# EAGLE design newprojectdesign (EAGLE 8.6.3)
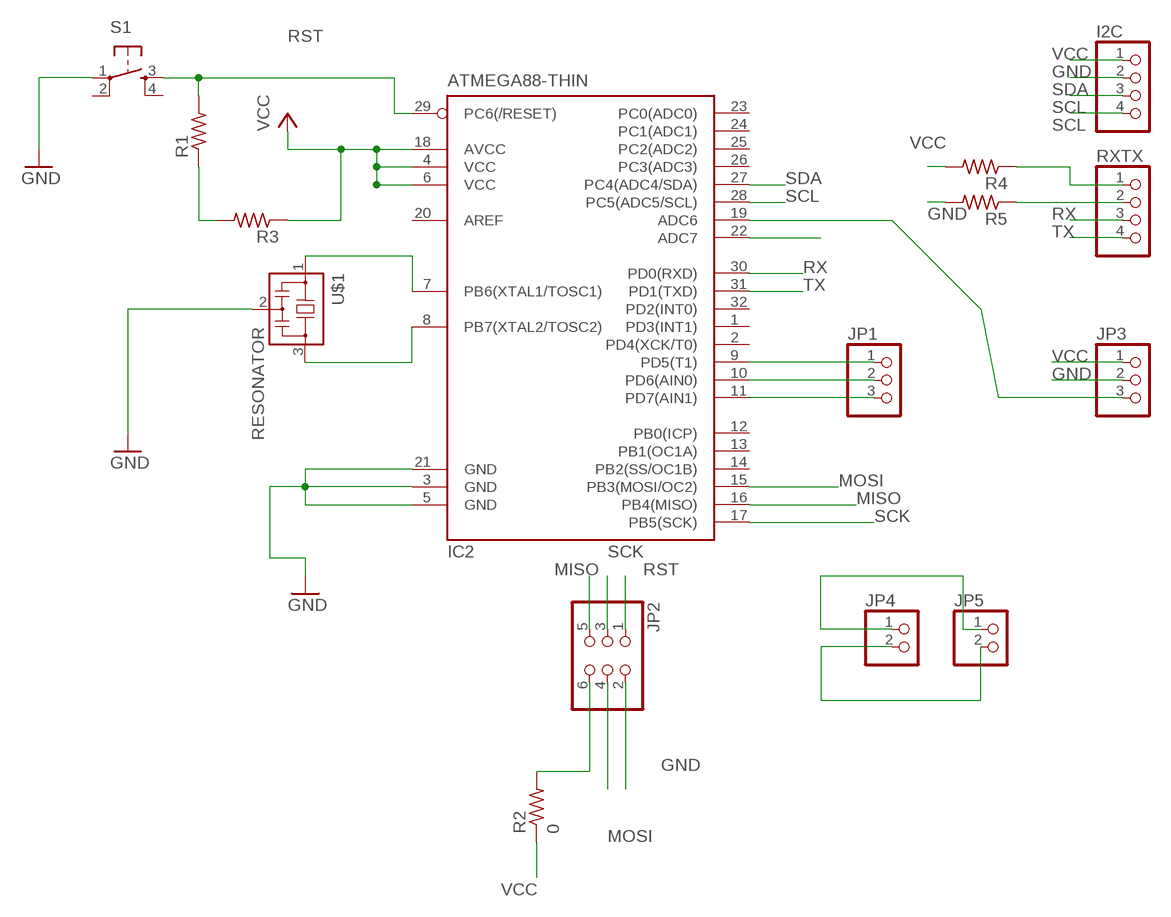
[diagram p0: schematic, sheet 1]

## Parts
I2C  PINHD-1X4  [1X04]
IC2  ATMEGA88-THIN  [TQFP32-08THIN]
JP1  PINHD-1X3  [1X03]
JP2  PINHD-2X3-SMD  [2X03SMD]
JP3  PINHD-1X3  [1X03]
JP4  PINHD-1X2  [1X02]
JP5  PINHD-1X2  [1X02]
R1  RES-US1206FAB  [R1206FAB]
R2  0  RES-US1206FAB  [R1206FAB]
R3  RES-US1206FAB  [R1206FAB]
R4  RES-US1206FAB  [R1206FAB]
R5  RES-US1206FAB  [R1206FAB]
RXTX  PINHD-1X4  [1X04]
S1  6MM_SWITCH6MM_SWITCH  [6MM_SWITCH]
U$1  RESONATOR  [EFOBM]

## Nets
GND: I2C.2 IC2.3(GND) IC2.5(GND) IC2.21(GND) JP2.2 JP3.2 JP4.2 JP5.2 R5.2 S1.1(P) U$1.2
MISO: IC2.16(PB4(MISO)) JP2.5
MOSI: IC2.15(PB3(MOSI/OC2)) JP2.4
N$1: R1.1 R3.2
N$2: IC2.9(PD5(T1)) JP1.1
N$3: JP2.6 R2.2
N$4: IC2.10(PD6(AIN0)) JP1.2
N$5: IC2.11(PD7(AIN1)) JP1.3
N$6: IC2.19(ADC6) JP3.3
N$7: IC2.22(ADC7)
N$8: IC2.8(PB7(XTAL2/TOSC2)) U$1.3
N$9: R4.1 RXTX.1
N$10: R5.1 RXTX.2
N$17: IC2.7(PB6(XTAL1/TOSC1)) U$1.1
RST: IC2.29(PC6(/RESET)) JP2.1 R1.2 S1.3(S)
RX: IC2.30(PD0(RXD)) RXTX.3
SCK: IC2.17(PB5(SCK)) JP2.3
SCL: I2C.4 IC2.28(PC5(ADC5/SCL))
SDA: I2C.3 IC2.27(PC4(ADC4/SDA))
TX: IC2.31(PD1(TXD)) RXTX.4
VCC: I2C.1 IC2.4(VCC) IC2.6(VCC) IC2.18(AVCC) JP3.1 JP4.1 JP5.1 R2.1 R3.1 R4.2
Unconnected: IC2.1(PD3(INT1)) IC2.2(PD4(XCK/T0)) IC2.12(PB0(ICP)) IC2.13(PB1(OC1A)) IC2.14(PB2(SS/OC1B)) IC2.20(AREF) IC2.23(PC0(ADC0)) IC2.24(PC1(ADC1)) IC2.25(PC2(ADC2)) IC2.26(PC3(ADC3)) IC2.32(PD2(INT0)) S1.2(P1) S1.4(S1)

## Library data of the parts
I2C RXTX = pinhead:PINHD-1X4: PIN HEADER
IC2 = fab:ATMEGA88-THIN
JP1 JP3 = adafruit:PINHD-1X3: PIN HEADER
JP2 = fab:PINHD-2X3-SMD: PIN HEADER
JP4 JP5 = pinhead:PINHD-1X2: PIN HEADER
R1-R5 = fab:RES-US: Resistor (US Symbol)
S1 = fab:6MM_SWITCH: OMRON SWITCH
U$1 = fab:RESONATOR

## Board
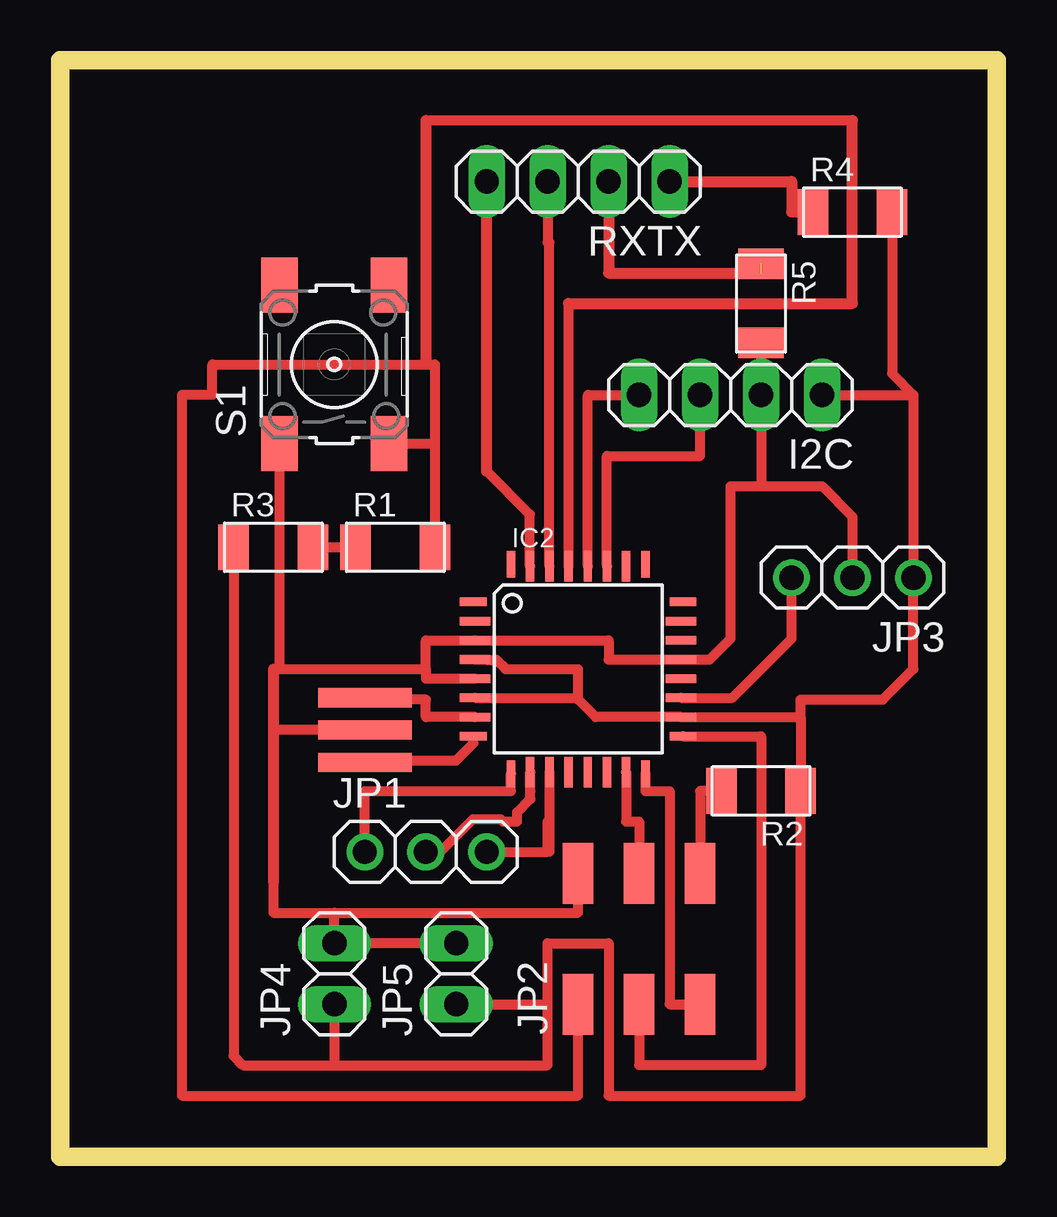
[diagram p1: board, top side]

Size 39.04 x 45.71 mm. Coordinates in mm from the lower left corner, seen from the top.
Outline: 0,0 39.04,0 39.04,45.71 0,45.71 0,0
Copper layers (1*16): Top 0.035mm / dielectric 1.5mm / Bottom 0.035mm
Design rules "default *": minimum track width 18mil, minimum drill 0.35mm, track to track 16mil, track to pad 16mil, pad to pad 16mil, via to via 16mil, smd to smd 16mil, copper to edge 40mil, drill to drill 6mil, minimum pad ring 10mil, minimum via ring 8mil, stop-mask expansion 4mil, vias tented up to drill 0mil, thermal gap 10mil

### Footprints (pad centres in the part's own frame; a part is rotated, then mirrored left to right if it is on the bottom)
1X04 = drill 1.016 long: 1 -3.81,0; 2 -1.27,0; 3 1.27,0; 4 3.81,0
TQFP32-08THIN = smd 1.118 x 0.356: 1 -4.369,2.8; 8 -4.369,-2.8; 17 4.369,-2.8; 24 4.369,2.8 | smd 1.27 x 0.356: 2 -4.293,2; 3 -4.293,1.2; 4 -4.293,0.4; 5 -4.293,-0.4; 6 -4.293,-1.2; 7 -4.293,-2; 18 4.293,-2; 19 4.293,-1.2; 20 4.293,-0.4; 21 4.293,0.4; 22 4.293,1.2; 23 4.293,2 | smd 0.356 x 1.118: 9 -2.8,-4.369; 16 2.8,-4.369; 25 2.8,4.369; 32 -2.8,4.369 | smd 0.356 x 1.27: 10 -2,-4.293; 14 1.2,-4.293; 15 2,-4.293; 26 2,4.293; 27 1.2,4.293; 31 -2,4.293 | smd 0.35 x 1.27: 11 -1.2,-4.293; 12 -0.4,-4.293; 13 0.4,-4.293; 28 0.4,4.293; 29 -0.4,4.293; 30 -1.2,4.293
1X03 = drill 1.016: 1 -2.54,0; 2 0,0; 3 2.54,0
2X03SMD = smd 2.54 x 1.27: 1 -2.54,2.54; 2 2.92,2.54; 3 -2.54,0; 4 2.92,0; 5 -2.54,-2.54; 6 2.92,-2.54
1X02 = drill 1.016 long: 1 -1.27,0; 2 1.27,0
R1206FAB = smd 1.27 x 1.905: 1 -1.651,0; 2 1.651,0
6MM_SWITCH = smd 2.286 x 1.524: 1 -3.302,2.286; 2 3.302,2.286; 3 -3.302,-2.286; 4 3.302,-2.286
EFOBM = smd 0.8 x 3.9: 1 -1.35,0; 2 0,0; 3 1.35,0

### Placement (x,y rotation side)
I2C  27.94,31.75 180 top
IC2  21.59,20.32 0 top
JP1  15.24,12.7 0 top
JP2  24.13,8.89 90 top
JP3  33.02,24.13 180 top
JP4  11.43,7.62 90 top
JP5  16.51,7.62 90 top
R1  13.97,25.4 0 top
R2  29.21,15.24 180 top
R3  8.89,25.4 0 top
R4  33.02,39.37 0 top
R5  29.21,35.56 270 top
RXTX  21.59,40.64 180 top
S1  11.43,33.02 90 top
U$1  12.7,17.78 270 top

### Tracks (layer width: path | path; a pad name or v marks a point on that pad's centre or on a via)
GND
  Top 0.406: IC2.5 15.24,19.92 15.24,20.32 | S1.1 9.14,20.32 | 9.14,20.32 8.89,20.32 | 9.14,20.32 15.24,20.32 | 15.24,20.32 15.24,21.52 IC2.3 22.86,21.52 22.86,20.72 IC2.21 27.07,20.72 27.94,21.59 27.94,27.94 29.21,27.94 | 29.21,27.94 I2C.2 R5.2 | 8.89,11.43 8.89,10.16 11.43,10.16 | JP2.2 21.59,10.16 11.43,10.16 | U$1.2 8.89,17.78 | 29.21,27.94 31.75,27.94 33.02,26.67 JP3.2 | 11.43,10.16 JP4.2 JP5.2
  Top 0.457: 8.89,20.32 8.89,17.78 8.89,11.43
MISO
  Top 0.406: IC2.16 24.39,15.24 25.4,15.24 25.4,6.35 JP2.5
MOSI
  Top 0.406: IC2.15 23.59,13.97 24.13,13.97 JP2.4
N$1
  Top 0.406: R3.2 R1.1
N$2
  Top 0.406: JP1.1 12.7,15.24 18.79,15.24 IC2.9
N$3
  Top 0.406: R2.2 26.67,15.24 JP2.6
N$4  (1 unrouted)
  Top 0.406: JP1.2 15.84,12.7 17.21,14.07 18.35,14.07 18.45,13.97 19.05,13.97 19.05,14.35 19.6,14.9 19.6,15.24 19.6,16.03
N$5
  Top 0.406: JP1.3 20.32,12.7 | 20.32,12.7 20.32,13.97 | IC2.11 20.39,12.7 20.32,12.7
N$6
  Top 0.406: IC2.19 28.01,19.12 30.48,21.59 JP3.3
N$8  (1 unrouted)
  Top 0.406: U$1.3 12.7,16.51 16.51,16.51 17.22,17.22 17.22,17.51
N$9
  Top 0.406: 30.48,39.37 R4.1
  Top 0.457: RXTX.1 30.48,40.64 30.48,39.37
N$10  (1 unrouted)
  Top 0.457: RXTX.2 22.86,36.83 29.21,36.83
N$17
  Top 0.406: U$1.1 12.7,19.05 15.24,19.05 15.24,18.32 IC2.7
RST
  Top 0.406: 15.62,29.72 R1.2 | IC2.29 21.19,35.56 | 33.02,43.18 15.24,43.18 | S1.3 15.62,29.72 | 15.62,29.72 15.62,33.02 15.24,33.02 6.35,33.02 6.35,31.75 5.08,31.75 5.08,2.54 21.59,2.54 JP2.1
  Top 0.457: 33.02,43.18 33.02,35.56 21.19,35.56 | 15.24,43.18 15.24,33.02
RX
  Top 0.406: IC2.30 20.39,38.1 20.32,38.1 RXTX.3
SCK
  Top 0.406: JP2.3 24.13,3.81 29.21,3.81 29.21,17.52 IC2.17
SCL
  Top 0.406: IC2.28 21.99,31.75 I2C.4
SDA
  Top 0.406: IC2.27 22.79,29.21 26.67,29.21 I2C.3
TX
  Top 0.406: IC2.31 19.58,24.62 19.58,26.77 17.78,28.57
  Top 0.457: 17.78,28.57 RXTX.4
VCC
  Top 0.406: 21.59,19.05 21.59,20.32 18.57,20.32 18.18,20.71 17.78,20.71 17.77,20.72 IC2.4 | 21.59,19.05 22.32,18.32 IC2.18 30.86,18.32 | IC2.6 21.52,19.12 21.59,19.05 | 30.86,18.32 R2.1 30.86,2.54 22.86,2.54 22.86,8.89 20.32,8.89 20.32,6.35 | R3.1 7.24,4.19 7.62,3.81 11.43,3.81 | 30.86,18.32 30.86,19.05 34.29,19.05 35.56,20.32 JP3.1 35.56,31.75 | I2C.1 35.56,31.75 | R4.2 34.67,32.64 35.56,31.75 | 11.43,3.81 20.32,3.81 20.32,6.35 | JP4.1 11.43,3.81 | JP5.1 20.32,6.35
